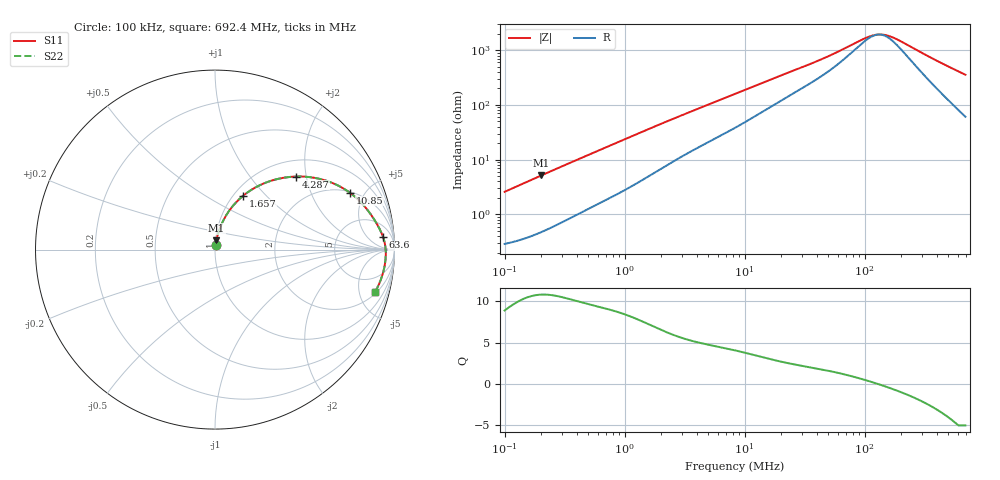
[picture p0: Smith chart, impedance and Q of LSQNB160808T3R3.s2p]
! LSQNB160808T3R3  S-PARAMETER MODEL  ( General Type )
! Model Generated by TAIYO YUDEN Corporation (http://www.ty-top.com)
! Version 2.0
! TAIYO YUDEN Control No. 100810NF25SB-FKC
! Copyright(c) 2007 TAIYO YUDEN CO.,LTD. All Rights Reserved.
! Product Description (link to TY-COMPAS)
! https://ds.yuden.co.jp/TYCOMPAS/or/detail?pn=LSQNB160808T3R3M&u=M
! Products Name : Inductors
! Characteristics :
!  Inductance : 3.3 uH , SRF(min) : 60 MHz , DC Resistance(max) : 0.286 Ohm
!  Rated Current : Saturation :170 mA , Temp Rise : 500 mA (40 degC)
!  Case Size : 1.6 x 0.8 / 0.063 x 0.031 [mm/inch] , Thickness : 0.8 / 0.031 [mm/inch]
!  (Conditions: Temperature = 25 degC , DC Bias Current/Voltage = 0A / 0V)
! External Node Assignments :
!  1  o---GGG---o  2
! GND o---------o GND
! Frequency Range : 0.1MHz  -  692.442054MHz  [ 402 STEP ]
# MHz S RI R 50
! Freq[MHz].  S11 Real  S11 Imag  S21 Real  S21 Imag  S12 Real  S12 Imag  S22 Real  S22 Imag
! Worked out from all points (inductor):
!   401 points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, 100 kHz to 692.4 MHz, reference 50 ohm
!   read as one part in series: L = 4.07 uH near 104.5 kHz
!   highest Q = 10.8 at 202.9 kHz (marker M1), where L = 4.03 uH
!   self-resonance near 130.1 MHz
!   S11 on the Smith chart (normalised r, x): 100 kHz: 1.01, +0.05; 1.657 MHz: 1.11, +0.75; 4.287 MHz: 1.35, +1.74; 10.85 MHz: 2.06, +3.91; 63.6 MHz: 13, +16; 692.4 MHz: 2.22, -7.02
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0.1  0.00353 0.0255  0.9965 -0.0255  0.9965 -0.0255  0.00353 0.0255
0.202876  0.00733 0.0508  0.9927 -0.0508  0.9927 -0.0508  0.00733 0.0508
0.439809  0.0219 0.1043  0.9781 -0.1043  0.9781 -0.1043  0.0219 0.1043
0.932603  0.0672 0.1988  0.9328 -0.1988  0.9328 -0.1988  0.0672 0.1988
1.656997  0.1563 0.2996  0.8437 -0.2996  0.8437 -0.2996  0.1563 0.2996
1.934321  0.1927 0.3265  0.8073 -0.3265  0.8073 -0.3265  0.1927 0.3265
2.94406  0.3175 0.385  0.6825 -0.385  0.6825 -0.385  0.3175 0.385
4.287094  0.4506 0.407  0.5494 -0.407  0.5494 -0.407  0.4506 0.407
5.972791  0.571 0.3966  0.429 -0.3966  0.429 -0.3966  0.571 0.3966
8.507318  0.6867 0.3564  0.3133 -0.3564  0.3133 -0.3564  0.6867 0.3564
10.84934  0.7513 0.317  0.2487 -0.317  0.2487 -0.317  0.7513 0.317
18.44277  0.8464 0.2251  0.1536 -0.2251  0.1536 -0.2251  0.8464 0.2251
36.59788  0.9093 0.13  0.0907 -0.13  0.0907 -0.13  0.9093 0.13
63.60334  0.9366 0.0695  0.0634 -0.0695  0.0634 -0.0695  0.9366 0.0695
96.80507  0.9474 0.0282  0.0526 -0.0282  0.0526 -0.0282  0.9474 0.0282
115.5329  0.9498 0.0114  0.0502 -0.0114  0.0502 -0.0114  0.9498 0.0114
134.8691  0.9511 -0.00342  0.0489 0.00342  0.0489 0.00342  0.9511 -0.00342
160.9608  0.9516 -0.0207  0.0484 0.0207  0.0484 0.0207  0.9516 -0.0207
196.3943  0.9511 -0.041  0.0489 0.041  0.0489 0.041  0.9511 -0.041
348.9424  0.9408 -0.1115  0.0592 0.1115  0.0592 0.1115  0.9408 -0.1115
531.0947  0.9185 -0.1812  0.0815 0.1812  0.0815 0.1812  0.9185 -0.1812
692.4421  0.892 -0.2356  0.108 0.2356  0.108 0.2356  0.892 -0.2356
